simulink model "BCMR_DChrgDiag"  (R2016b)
settings: Solver=FixedStepDiscrete  StartTime=0.0  StopTime=10  FixedStep=0.01  RelTol=1e-3  EnableMultiTasking=on
undefined symbols (not defined in the file or in its folder): BCMR_bDChrgStopCActiveSw_C, BCMR_cntDChrgTCnntMax_C, BCMR_cntIsoFltTrigger_CW, BCMR_EVCCDiagccSw_C, BCMR_EVCCDiagSw_C, BCMR_G1E0PlatformSwDiag_C, BCMR_H1U0PlatformSwDiag_C, BCMR_iDcChrgDiffOvrCurr_C, BCMR_iDcChrgLowTempDiffOvrCurrMody_C, BCMR_iDcChrgLowTempOvrCurrCutOff_C, BCMR_iDcChrgLowTempOvrCurrHeal_C, BCMR_iDcChrgOvrCurr_C, BCMR_iDcChrgOvrVolt_C, BCMR_iDChrgCurrDiagLmt_C, BCMR_iDChrgCutOffVoltOvrCurrDet_C, BCMR_iDChrgCutOffVoltOvrCurrHeal_C, BCMR_kWaveFltFactor_C, BCMR_stCCSTimeout_C, BCMR_stCHMTimeout_C, BCMR_stCMLTimeout_C, BCMR_stCRMAATimeout_C, BCMR_stCROAATimeout_C, BCMR_stCROTimeout_C, BCMR_stCSDTimeout1_C, BCMR_stCSDTimeout2_C, BCMR_stCSTTimeout_C, BCMR_stCurrDwnTimeout_C, BCMR_stHvOnTimeout_C, BCMR_stNoTimeout_C, BCMR_stParaMish_C, BCMR_tBattLowTempDiagTempThrd_C, BCMR_tDcChrgIntfTempDiffLmt_C, BCMR_tDcChrgIntfTempLmt_C, BCMR_tiDChrgDetDiagDebs_C, BCMR_tiDChrgDetSec_C, BCMR_tiDChrgDiagBase_C, BCMR_tiDChrgHealDiagDebs_C, BCMR_tiDChrgIntfTempDwnLmt_C, BCMR_tiDChrgLowTOvrCurrDet_C, BCMR_tiDChrgLowTOvrCurrHeal_C, BCMR_tiDChrgMishCurrDetDiagDebs_C, BCMR_tiDChrgOvrCellVolt_C, BCMR_tiDChrgOvrSafeCellVoltDet_C, BCMR_tiDChrgVoltFltDetDebs_C, BCMR_tiDChrgVoltFltHealDebs_C, BCMR_uCC2ChkDiffDet_C, BCMR_uCC2ChkDiffHeal_C, BCMR_uCC2VoltHighDet_C, BCMR_uCC2VoltHighHeal_C, BCMR_uCC2VoltLowDet_C, BCMR_uCC2VoltLowHeal_C, BCMR_uDChrgHighTempDet_C, BCMR_uDChrgHighTempHeal_C, BCMR_uDChrgLowTempDet_C, BCMR_uDChrgLowTempHeal_C, BCMR_uDChrgOvrCellVoltDet_C, BCMR_uDChrgOvrCellVoltHeal_C, BCMR_uDChrgOvrSafeCellVoltDet_C, BCMR_uDChrgOvrSafeCellVoltHeal_C, bin2dec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
libraries: simulink x291
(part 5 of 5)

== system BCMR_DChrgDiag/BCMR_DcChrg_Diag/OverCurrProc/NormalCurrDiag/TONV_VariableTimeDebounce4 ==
  note: Turn On Delay Time Deboune
  u : Inport
  T : Inport  Port=2
  dT : Inport  Port=3
  Add : Sum
  Constant1 : Constant  Value=0  OutDataTypeStr=single
  Constant2 : Constant  OutDataTypeStr=uint8
  Constant3 : Constant  Value=0  OutDataTypeStr=uint8
  Delay : Delay  DelayLength=1  InitialCondition=0
  MinMax : MinMax  Inputs=2
  Product : Product  OutMin=[0]  OutMax=[65535]  OutDataTypeStr=single
  Relational Operator : RelationalOperator  Operator=>  OutDataTypeStr=boolean  RndMeth=Simplest
  Switch : Switch  Criteria=u2 ~= 0
  Switch1 : Switch  Criteria=u2 ~= 0
  y : Outport
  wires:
  Switch1/1 -> Product/1
  Constant3/1 -> Switch1/3
  Constant2/1 -> Switch1/1
  u/1 -> Switch1/2, Switch/2
  dT/1 -> Switch/1
  Constant1/1 -> Switch/3
  Add/1 -> Product/2
  Product/1 -> Relational Operator/1, Delay/1
  Switch/1 -> Add/1
  Delay/1 -> MinMax/2
  Relational Operator/1 -> y/1
  T/1 -> MinMax/1, Relational Operator/2
  MinMax/1 -> Add/2

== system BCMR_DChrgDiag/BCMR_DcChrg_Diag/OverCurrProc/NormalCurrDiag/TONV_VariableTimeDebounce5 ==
  note: Turn On Delay Time Deboune
  u : Inport
  T : Inport  Port=2
  dT : Inport  Port=3
  Add : Sum
  Constant1 : Constant  Value=0  OutDataTypeStr=single
  Constant2 : Constant  OutDataTypeStr=uint8
  Constant3 : Constant  Value=0  OutDataTypeStr=uint8
  Delay : Delay  DelayLength=1  InitialCondition=0
  MinMax : MinMax  Inputs=2
  Product : Product  OutMin=[0]  OutMax=[65535]  OutDataTypeStr=single
  Relational Operator : RelationalOperator  Operator=>  OutDataTypeStr=boolean  RndMeth=Simplest
  Switch : Switch  Criteria=u2 ~= 0
  Switch1 : Switch  Criteria=u2 ~= 0
  y : Outport
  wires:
  Switch1/1 -> Product/1
  Constant3/1 -> Switch1/3
  Constant2/1 -> Switch1/1
  u/1 -> Switch1/2, Switch/2
  dT/1 -> Switch/1
  Constant1/1 -> Switch/3
  Add/1 -> Product/2
  Product/1 -> Relational Operator/1, Delay/1
  Switch/1 -> Add/1
  Delay/1 -> MinMax/2
  Relational Operator/1 -> y/1
  T/1 -> MinMax/1, Relational Operator/2
  MinMax/1 -> Add/2

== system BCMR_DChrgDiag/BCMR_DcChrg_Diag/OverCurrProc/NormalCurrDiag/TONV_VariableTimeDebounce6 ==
  note: Turn On Delay Time Deboune
  u : Inport
  T : Inport  Port=2
  dT : Inport  Port=3
  Add : Sum
  Constant1 : Constant  Value=0  OutDataTypeStr=single
  Constant2 : Constant  OutDataTypeStr=uint8
  Constant3 : Constant  Value=0  OutDataTypeStr=uint8
  Delay : Delay  DelayLength=1  InitialCondition=0
  MinMax : MinMax  Inputs=2
  Product : Product  OutMin=[0]  OutMax=[65535]  OutDataTypeStr=single
  Relational Operator : RelationalOperator  Operator=>  OutDataTypeStr=boolean  RndMeth=Simplest
  Switch : Switch  Criteria=u2 ~= 0
  Switch1 : Switch  Criteria=u2 ~= 0
  y : Outport
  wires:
  Switch1/1 -> Product/1
  Constant3/1 -> Switch1/3
  Constant2/1 -> Switch1/1
  u/1 -> Switch1/2, Switch/2
  dT/1 -> Switch/1
  Constant1/1 -> Switch/3
  Add/1 -> Product/2
  Product/1 -> Relational Operator/1, Delay/1
  Switch/1 -> Add/1
  Delay/1 -> MinMax/2
  Relational Operator/1 -> y/1
  T/1 -> MinMax/1, Relational Operator/2
  MinMax/1 -> Add/2

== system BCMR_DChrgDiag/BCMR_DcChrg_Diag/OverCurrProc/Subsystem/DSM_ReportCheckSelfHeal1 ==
  note: Fault report to diagnostic management system
  Dfc_id_nv : Inport  OutDataTypeStr=uint8
  Err : Inport  Port=2
  Heal : Inport  Port=3
  Bit Clear1 : simulink/Logic and Bit Operations/Bit Clear  iBit=4
  Bit Clear2 : simulink/Logic and Bit Operations/Bit Clear  iBit=3
  Bit Set : simulink/Logic and Bit Operations/Bit Set  iBit=4
  Bit Set1 : simulink/Logic and Bit Operations/Bit Set  iBit=3
  Bit Set2 : simulink/Logic and Bit Operations/Bit Set  iBit=3
  Bit Set4 : simulink/Logic and Bit Operations/Bit Set  iBit=7
  Constant1 : Constant  Value=0  OutDataTypeStr=uint8
  Constant7 : Constant  Value=0  OutDataTypeStr=boolean
  Delay2 : Delay  DelayLength=1  InitialCondition=1
  Delay3 : Delay  DelayLength=1  InitialCondition=0
  Logical Operator : Logic  Operator=OR  AllPortsSameDT=off  OutDataTypeStr=boolean
  Switch{1..4} (4 alike) : Switch  Criteria=u2 ~= 0
  Dfc_id : Outport  OutDataTypeStr=uint8
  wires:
  Dfc_id_nv/1 -> Bit Clear2/1, Bit Set4/1, Bit Clear1/1
  Bit Set4/1 -> Bit Set/1
  Constant7/1 -> Delay2/1
  Delay2/1 -> Switch2/2
  Switch3/1 -> Switch2/3
  Bit Clear2/1 -> Switch2/1
  Switch2/1 -> Delay3/1, Switch1/1
  Bit Set1/1 -> Switch3/1
  Bit Set/1 -> Bit Set1/1
  Switch4/1 -> Switch3/3
  Err/1 -> Logical Operator/2, Switch3/2
  Bit Set2/1 -> Switch4/1
  Bit Clear1/1 -> Bit Set2/1
  Delay3/1 -> Switch4/3
  Heal/1 -> Logical Operator/1, Switch4/2
  Logical Operator/1 -> Switch1/2
  Constant1/1 -> Switch1/3
  Switch1/1 -> Dfc_id/1

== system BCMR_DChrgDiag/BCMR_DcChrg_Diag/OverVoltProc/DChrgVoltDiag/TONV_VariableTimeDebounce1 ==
  note: Turn On Delay Time Deboune
  u : Inport
  T : Inport  Port=2
  dT : Inport  Port=3
  Add : Sum
  Constant1 : Constant  Value=0  OutDataTypeStr=single
  Constant2 : Constant  OutDataTypeStr=uint8
  Constant3 : Constant  Value=0  OutDataTypeStr=uint8
  Delay : Delay  DelayLength=1  InitialCondition=0
  MinMax : MinMax  Inputs=2
  Product : Product  OutMin=[0]  OutMax=[65535]  OutDataTypeStr=single
  Relational Operator : RelationalOperator  Operator=>  OutDataTypeStr=boolean  RndMeth=Simplest
  Switch : Switch  Criteria=u2 ~= 0
  Switch1 : Switch  Criteria=u2 ~= 0
  y : Outport
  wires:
  Switch1/1 -> Product/1
  Constant3/1 -> Switch1/3
  Constant2/1 -> Switch1/1
  u/1 -> Switch1/2, Switch/2
  dT/1 -> Switch/1
  Constant1/1 -> Switch/3
  Add/1 -> Product/2
  Product/1 -> Relational Operator/1, Delay/1
  Switch/1 -> Add/1
  Delay/1 -> MinMax/2
  Relational Operator/1 -> y/1
  T/1 -> MinMax/1, Relational Operator/2
  MinMax/1 -> Add/2

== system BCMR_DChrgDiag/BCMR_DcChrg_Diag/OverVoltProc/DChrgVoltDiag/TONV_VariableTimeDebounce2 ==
  note: Turn On Delay Time Deboune
  u : Inport
  T : Inport  Port=2
  dT : Inport  Port=3
  Add : Sum
  Constant1 : Constant  Value=0  OutDataTypeStr=single
  Constant2 : Constant  OutDataTypeStr=uint8
  Constant3 : Constant  Value=0  OutDataTypeStr=uint8
  Delay : Delay  DelayLength=1  InitialCondition=0
  MinMax : MinMax  Inputs=2
  Product : Product  OutMin=[0]  OutMax=[65535]  OutDataTypeStr=single
  Relational Operator : RelationalOperator  Operator=>  OutDataTypeStr=boolean  RndMeth=Simplest
  Switch : Switch  Criteria=u2 ~= 0
  Switch1 : Switch  Criteria=u2 ~= 0
  y : Outport
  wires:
  Switch1/1 -> Product/1
  Constant3/1 -> Switch1/3
  Constant2/1 -> Switch1/1
  u/1 -> Switch1/2, Switch/2
  dT/1 -> Switch/1
  Constant1/1 -> Switch/3
  Add/1 -> Product/2
  Product/1 -> Relational Operator/1, Delay/1
  Switch/1 -> Add/1
  Delay/1 -> MinMax/2
  Relational Operator/1 -> y/1
  T/1 -> MinMax/1, Relational Operator/2
  MinMax/1 -> Add/2

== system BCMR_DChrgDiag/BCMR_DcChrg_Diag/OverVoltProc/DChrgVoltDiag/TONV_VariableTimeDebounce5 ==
  note: Turn On Delay Time Deboune
  u : Inport
  T : Inport  Port=2
  dT : Inport  Port=3
  Add : Sum
  Constant1 : Constant  Value=0  OutDataTypeStr=single
  Constant2 : Constant  OutDataTypeStr=uint8
  Constant3 : Constant  Value=0  OutDataTypeStr=uint8
  Delay : Delay  DelayLength=1  InitialCondition=0
  MinMax : MinMax  Inputs=2
  Product : Product  OutMin=[0]  OutMax=[65535]  OutDataTypeStr=single
  Relational Operator : RelationalOperator  Operator=>  OutDataTypeStr=boolean  RndMeth=Simplest
  Switch : Switch  Criteria=u2 ~= 0
  Switch1 : Switch  Criteria=u2 ~= 0
  y : Outport
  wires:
  Switch1/1 -> Product/1
  Constant3/1 -> Switch1/3
  Constant2/1 -> Switch1/1
  u/1 -> Switch1/2, Switch/2
  dT/1 -> Switch/1
  Constant1/1 -> Switch/3
  Add/1 -> Product/2
  Product/1 -> Relational Operator/1, Delay/1
  Switch/1 -> Add/1
  Delay/1 -> MinMax/2
  Relational Operator/1 -> y/1
  T/1 -> MinMax/1, Relational Operator/2
  MinMax/1 -> Add/2

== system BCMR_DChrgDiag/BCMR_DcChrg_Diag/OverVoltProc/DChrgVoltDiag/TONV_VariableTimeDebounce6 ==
  note: Turn On Delay Time Deboune
  u : Inport
  T : Inport  Port=2
  dT : Inport  Port=3
  Add : Sum
  Constant1 : Constant  Value=0  OutDataTypeStr=single
  Constant2 : Constant  OutDataTypeStr=uint8
  Constant3 : Constant  Value=0  OutDataTypeStr=uint8
  Delay : Delay  DelayLength=1  InitialCondition=0
  MinMax : MinMax  Inputs=2
  Product : Product  OutMin=[0]  OutMax=[65535]  OutDataTypeStr=single
  Relational Operator : RelationalOperator  Operator=>  OutDataTypeStr=boolean  RndMeth=Simplest
  Switch : Switch  Criteria=u2 ~= 0
  Switch1 : Switch  Criteria=u2 ~= 0
  y : Outport
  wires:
  Switch1/1 -> Product/1
  Constant3/1 -> Switch1/3
  Constant2/1 -> Switch1/1
  u/1 -> Switch1/2, Switch/2
  dT/1 -> Switch/1
  Constant1/1 -> Switch/3
  Add/1 -> Product/2
  Product/1 -> Relational Operator/1, Delay/1
  Switch/1 -> Add/1
  Delay/1 -> MinMax/2
  Relational Operator/1 -> y/1
  T/1 -> MinMax/1, Relational Operator/2
  MinMax/1 -> Add/2

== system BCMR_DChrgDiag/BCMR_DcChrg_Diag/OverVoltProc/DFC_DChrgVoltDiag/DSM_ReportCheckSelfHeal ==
  note: Fault report to diagnostic management system
  Dfc_id_nv : Inport  OutDataTypeStr=uint8
  Err : Inport  Port=2
  Heal : Inport  Port=3
  Bit Clear1 : simulink/Logic and Bit Operations/Bit Clear  iBit=4
  Bit Clear2 : simulink/Logic and Bit Operations/Bit Clear  iBit=3
  Bit Set : simulink/Logic and Bit Operations/Bit Set  iBit=4
  Bit Set1 : simulink/Logic and Bit Operations/Bit Set  iBit=3
  Bit Set2 : simulink/Logic and Bit Operations/Bit Set  iBit=3
  Bit Set4 : simulink/Logic and Bit Operations/Bit Set  iBit=7
  Constant1 : Constant  Value=0  OutDataTypeStr=uint8
  Constant7 : Constant  Value=0  OutDataTypeStr=boolean
  Delay2 : Delay  DelayLength=1  InitialCondition=1
  Delay3 : Delay  DelayLength=1  InitialCondition=0
  Logical Operator : Logic  Operator=OR  AllPortsSameDT=off  OutDataTypeStr=boolean
  Switch{1..4} (4 alike) : Switch  Criteria=u2 ~= 0
  Dfc_id : Outport  OutDataTypeStr=uint8
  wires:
  Dfc_id_nv/1 -> Bit Clear2/1, Bit Set4/1, Bit Clear1/1
  Bit Set4/1 -> Bit Set/1
  Constant7/1 -> Delay2/1
  Delay2/1 -> Switch2/2
  Switch3/1 -> Switch2/3
  Bit Clear2/1 -> Switch2/1
  Switch2/1 -> Delay3/1, Switch1/1
  Bit Set1/1 -> Switch3/1
  Bit Set/1 -> Bit Set1/1
  Switch4/1 -> Switch3/3
  Err/1 -> Logical Operator/2, Switch3/2
  Bit Set2/1 -> Switch4/1
  Bit Clear1/1 -> Bit Set2/1
  Delay3/1 -> Switch4/3
  Heal/1 -> Logical Operator/1, Switch4/2
  Logical Operator/1 -> Switch1/2
  Constant1/1 -> Switch1/3
  Switch1/1 -> Dfc_id/1

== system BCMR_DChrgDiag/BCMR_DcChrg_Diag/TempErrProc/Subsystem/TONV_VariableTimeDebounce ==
  note: Turn On Delay Time Deboune
  u : Inport
  T : Inport  Port=2
  dT : Inport  Port=3
  Add : Sum
  Constant1 : Constant  Value=0  OutDataTypeStr=single
  Constant2 : Constant  OutDataTypeStr=uint8
  Constant3 : Constant  Value=0  OutDataTypeStr=uint8
  Delay : Delay  DelayLength=1  InitialCondition=0
  MinMax : MinMax  Inputs=2
  Product : Product  OutMin=[0]  OutMax=[65535]  OutDataTypeStr=single
  Relational Operator : RelationalOperator  Operator=>  OutDataTypeStr=boolean  RndMeth=Simplest
  Switch : Switch  Criteria=u2 ~= 0
  Switch1 : Switch  Criteria=u2 ~= 0
  y : Outport
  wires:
  Switch1/1 -> Product/1
  Constant3/1 -> Switch1/3
  Constant2/1 -> Switch1/1
  u/1 -> Switch1/2, Switch/2
  dT/1 -> Switch/1
  Constant1/1 -> Switch/3
  Add/1 -> Product/2
  Product/1 -> Relational Operator/1, Delay/1
  Switch/1 -> Add/1
  Delay/1 -> MinMax/2
  Relational Operator/1 -> y/1
  T/1 -> MinMax/1, Relational Operator/2
  MinMax/1 -> Add/2

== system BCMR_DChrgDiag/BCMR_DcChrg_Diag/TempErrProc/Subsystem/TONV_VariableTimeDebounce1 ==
  note: Turn On Delay Time Deboune
  u : Inport
  T : Inport  Port=2
  dT : Inport  Port=3
  Add : Sum
  Constant1 : Constant  Value=0  OutDataTypeStr=single
  Constant2 : Constant  OutDataTypeStr=uint8
  Constant3 : Constant  Value=0  OutDataTypeStr=uint8
  Delay : Delay  DelayLength=1  InitialCondition=0
  MinMax : MinMax  Inputs=2
  Product : Product  OutMin=[0]  OutMax=[65535]  OutDataTypeStr=single
  Relational Operator : RelationalOperator  Operator=>  OutDataTypeStr=boolean  RndMeth=Simplest
  Switch : Switch  Criteria=u2 ~= 0
  Switch1 : Switch  Criteria=u2 ~= 0
  y : Outport
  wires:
  Switch1/1 -> Product/1
  Constant3/1 -> Switch1/3
  Constant2/1 -> Switch1/1
  u/1 -> Switch1/2, Switch/2
  dT/1 -> Switch/1
  Constant1/1 -> Switch/3
  Add/1 -> Product/2
  Product/1 -> Relational Operator/1, Delay/1
  Switch/1 -> Add/1
  Delay/1 -> MinMax/2
  Relational Operator/1 -> y/1
  T/1 -> MinMax/1, Relational Operator/2
  MinMax/1 -> Add/2

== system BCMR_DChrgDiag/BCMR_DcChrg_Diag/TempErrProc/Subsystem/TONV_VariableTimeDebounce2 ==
  note: Turn On Delay Time Deboune
  u : Inport
  T : Inport  Port=2
  dT : Inport  Port=3
  Add : Sum
  Constant1 : Constant  Value=0  OutDataTypeStr=single
  Constant2 : Constant  OutDataTypeStr=uint8
  Constant3 : Constant  Value=0  OutDataTypeStr=uint8
  Delay : Delay  DelayLength=1  InitialCondition=0
  MinMax : MinMax  Inputs=2
  Product : Product  OutMin=[0]  OutMax=[65535]  OutDataTypeStr=single
  Relational Operator : RelationalOperator  Operator=>  OutDataTypeStr=boolean  RndMeth=Simplest
  Switch : Switch  Criteria=u2 ~= 0
  Switch1 : Switch  Criteria=u2 ~= 0
  y : Outport
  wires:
  MinMax/1 -> Add/2
  T/1 -> Relational Operator/2, MinMax/1
  Relational Operator/1 -> y/1
  Delay/1 -> MinMax/2
  Switch/1 -> Add/1
  Product/1 -> Delay/1, Relational Operator/1
  Add/1 -> Product/2
  Constant1/1 -> Switch/3
  dT/1 -> Switch/1
  u/1 -> Switch/2, Switch1/2
  Constant2/1 -> Switch1/1
  Constant3/1 -> Switch1/3
  Switch1/1 -> Product/1

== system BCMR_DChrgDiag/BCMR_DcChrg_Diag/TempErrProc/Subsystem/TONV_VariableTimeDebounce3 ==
  note: Turn On Delay Time Deboune
  u : Inport
  T : Inport  Port=2
  dT : Inport  Port=3
  Add : Sum
  Constant1 : Constant  Value=0  OutDataTypeStr=single
  Constant2 : Constant  OutDataTypeStr=uint8
  Constant3 : Constant  Value=0  OutDataTypeStr=uint8
  Delay : Delay  DelayLength=1  InitialCondition=0
  MinMax : MinMax  Inputs=2
  Product : Product  OutMin=[0]  OutMax=[65535]  OutDataTypeStr=single
  Relational Operator : RelationalOperator  Operator=>  OutDataTypeStr=boolean  RndMeth=Simplest
  Switch : Switch  Criteria=u2 ~= 0
  Switch1 : Switch  Criteria=u2 ~= 0
  y : Outport
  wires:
  MinMax/1 -> Add/2
  T/1 -> Relational Operator/2, MinMax/1
  Relational Operator/1 -> y/1
  Delay/1 -> MinMax/2
  Switch/1 -> Add/1
  Product/1 -> Delay/1, Relational Operator/1
  Add/1 -> Product/2
  Constant1/1 -> Switch/3
  dT/1 -> Switch/1
  u/1 -> Switch/2, Switch1/2
  Constant2/1 -> Switch1/1
  Constant3/1 -> Switch1/3
  Switch1/1 -> Product/1

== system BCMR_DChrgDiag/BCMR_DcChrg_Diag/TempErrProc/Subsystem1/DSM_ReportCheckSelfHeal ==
  note: Fault report to diagnostic management system
  Dfc_id_nv : Inport  OutDataTypeStr=uint8
  Err : Inport  Port=2
  Heal : Inport  Port=3
  Bit Clear1 : simulink/Logic and Bit Operations/Bit Clear  iBit=4
  Bit Clear2 : simulink/Logic and Bit Operations/Bit Clear  iBit=3
  Bit Set : simulink/Logic and Bit Operations/Bit Set  iBit=4
  Bit Set1 : simulink/Logic and Bit Operations/Bit Set  iBit=3
  Bit Set2 : simulink/Logic and Bit Operations/Bit Set  iBit=3
  Bit Set4 : simulink/Logic and Bit Operations/Bit Set  iBit=7
  Constant1 : Constant  Value=0  OutDataTypeStr=uint8
  Constant7 : Constant  Value=0  OutDataTypeStr=boolean
  Delay2 : Delay  DelayLength=1  InitialCondition=1
  Delay3 : Delay  DelayLength=1  InitialCondition=0
  Logical Operator : Logic  Operator=OR  AllPortsSameDT=off  OutDataTypeStr=boolean
  Switch{1..4} (4 alike) : Switch  Criteria=u2 ~= 0
  Dfc_id : Outport  OutDataTypeStr=uint8
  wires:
  Dfc_id_nv/1 -> Bit Clear2/1, Bit Set4/1, Bit Clear1/1
  Bit Set4/1 -> Bit Set/1
  Constant7/1 -> Delay2/1
  Delay2/1 -> Switch2/2
  Switch3/1 -> Switch2/3
  Bit Clear2/1 -> Switch2/1
  Switch2/1 -> Delay3/1, Switch1/1
  Bit Set1/1 -> Switch3/1
  Bit Set/1 -> Bit Set1/1
  Switch4/1 -> Switch3/3
  Err/1 -> Logical Operator/2, Switch3/2
  Bit Set2/1 -> Switch4/1
  Bit Clear1/1 -> Bit Set2/1
  Delay3/1 -> Switch4/3
  Heal/1 -> Logical Operator/1, Switch4/2
  Logical Operator/1 -> Switch1/2
  Constant1/1 -> Switch1/3
  Switch1/1 -> Dfc_id/1

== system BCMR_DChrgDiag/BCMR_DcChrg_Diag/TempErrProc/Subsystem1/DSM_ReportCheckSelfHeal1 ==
  note: Fault report to diagnostic management system
  Dfc_id_nv : Inport  OutDataTypeStr=uint8
  Err : Inport  Port=2
  Heal : Inport  Port=3
  Bit Clear1 : simulink/Logic and Bit Operations/Bit Clear  iBit=4
  Bit Clear2 : simulink/Logic and Bit Operations/Bit Clear  iBit=3
  Bit Set : simulink/Logic and Bit Operations/Bit Set  iBit=4
  Bit Set1 : simulink/Logic and Bit Operations/Bit Set  iBit=3
  Bit Set2 : simulink/Logic and Bit Operations/Bit Set  iBit=3
  Bit Set4 : simulink/Logic and Bit Operations/Bit Set  iBit=7
  Constant1 : Constant  Value=0  OutDataTypeStr=uint8
  Constant7 : Constant  Value=0  OutDataTypeStr=boolean
  Delay2 : Delay  DelayLength=1  InitialCondition=1
  Delay3 : Delay  DelayLength=1  InitialCondition=0
  Logical Operator : Logic  Operator=OR  AllPortsSameDT=off  OutDataTypeStr=boolean
  Switch{1..4} (4 alike) : Switch  Criteria=u2 ~= 0
  Dfc_id : Outport  OutDataTypeStr=uint8
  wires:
  Switch1/1 -> Dfc_id/1
  Constant1/1 -> Switch1/3
  Logical Operator/1 -> Switch1/2
  Heal/1 -> Switch4/2, Logical Operator/1
  Delay3/1 -> Switch4/3
  Bit Clear1/1 -> Bit Set2/1
  Bit Set2/1 -> Switch4/1
  Err/1 -> Switch3/2, Logical Operator/2
  Switch4/1 -> Switch3/3
  Bit Set/1 -> Bit Set1/1
  Bit Set1/1 -> Switch3/1
  Switch2/1 -> Switch1/1, Delay3/1
  Bit Clear2/1 -> Switch2/1
  Switch3/1 -> Switch2/3
  Delay2/1 -> Switch2/2
  Constant7/1 -> Delay2/1
  Bit Set4/1 -> Bit Set/1
  Dfc_id_nv/1 -> Bit Clear1/1, Bit Set4/1, Bit Clear2/1

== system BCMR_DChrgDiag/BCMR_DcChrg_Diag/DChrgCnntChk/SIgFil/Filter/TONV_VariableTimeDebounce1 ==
  note: Turn On Delay Time Deboune
  u : Inport
  T : Inport  Port=2
  dT : Inport  Port=3
  Add : Sum
  Constant1 : Constant  Value=0  OutDataTypeStr=single
  Constant2 : Constant  OutDataTypeStr=uint8
  Constant3 : Constant  Value=0  OutDataTypeStr=uint8
  Delay : Delay  DelayLength=1  InitialCondition=0
  MinMax : MinMax  Inputs=2
  Product : Product  OutMin=[0]  OutMax=[65535]  OutDataTypeStr=single
  Relational Operator : RelationalOperator  Operator=>  OutDataTypeStr=boolean  RndMeth=Simplest
  Switch : Switch  Criteria=u2 ~= 0
  Switch1 : Switch  Criteria=u2 ~= 0
  y : Outport
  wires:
  Switch1/1 -> Product/1
  Constant3/1 -> Switch1/3
  Constant2/1 -> Switch1/1
  u/1 -> Switch1/2, Switch/2
  dT/1 -> Switch/1
  Constant1/1 -> Switch/3
  Add/1 -> Product/2
  Product/1 -> Relational Operator/1, Delay/1
  Switch/1 -> Add/1
  Delay/1 -> MinMax/2
  Relational Operator/1 -> y/1
  T/1 -> MinMax/1, Relational Operator/2
  MinMax/1 -> Add/2

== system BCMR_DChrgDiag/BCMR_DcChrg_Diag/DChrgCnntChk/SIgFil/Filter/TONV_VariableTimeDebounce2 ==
  note: Turn On Delay Time Deboune
  u : Inport
  T : Inport  Port=2
  dT : Inport  Port=3
  Add : Sum
  Constant1 : Constant  Value=0  OutDataTypeStr=single
  Constant2 : Constant  OutDataTypeStr=uint8
  Constant3 : Constant  Value=0  OutDataTypeStr=uint8
  Delay : Delay  DelayLength=1  InitialCondition=0
  MinMax : MinMax  Inputs=2
  Product : Product  OutMin=[0]  OutMax=[65535]  OutDataTypeStr=single
  Relational Operator : RelationalOperator  Operator=>  OutDataTypeStr=boolean  RndMeth=Simplest
  Switch : Switch  Criteria=u2 ~= 0
  Switch1 : Switch  Criteria=u2 ~= 0
  y : Outport
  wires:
  Switch1/1 -> Product/1
  Constant3/1 -> Switch1/3
  Constant2/1 -> Switch1/1
  u/1 -> Switch1/2, Switch/2
  dT/1 -> Switch/1
  Constant1/1 -> Switch/3
  Add/1 -> Product/2
  Product/1 -> Relational Operator/1, Delay/1
  Switch/1 -> Add/1
  Delay/1 -> MinMax/2
  Relational Operator/1 -> y/1
  T/1 -> MinMax/1, Relational Operator/2
  MinMax/1 -> Add/2

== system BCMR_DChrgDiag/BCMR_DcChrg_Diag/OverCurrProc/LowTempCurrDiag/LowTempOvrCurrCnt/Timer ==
  En : Inport
  Cnt : Inport  Port=2
  Rst : Inport  Port=3
  Vst : Inport  Port=4
  Add : Sum
  Constant5 : Constant  Value=single(0)  OutDataTypeStr=single
  Switch1 : Switch  Criteria=u2 ~= 0
  Switch2 : Switch  Criteria=u2 ~= 0
  Unit Delay : UnitDelay  SampleTime=-1
  Number : Outport
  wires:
  Unit Delay/1 -> Add/2
  Rst/1 -> Switch1/2
  En/1 -> Switch2/2
  Cnt/1 -> Switch2/1
  Constant5/1 -> Switch2/3
  Switch2/1 -> Add/1
  Vst/1 -> Switch1/1
  Switch1/1 -> Number/1, Unit Delay/1
  Add/1 -> Switch1/3
